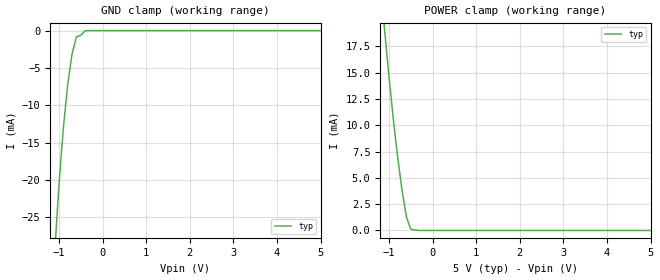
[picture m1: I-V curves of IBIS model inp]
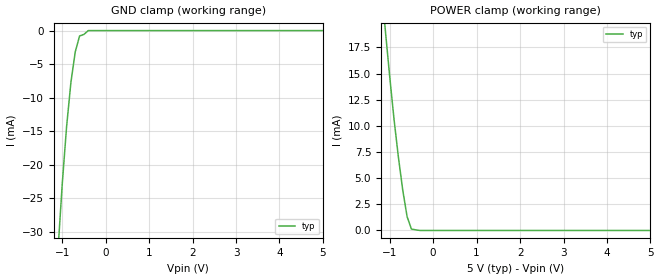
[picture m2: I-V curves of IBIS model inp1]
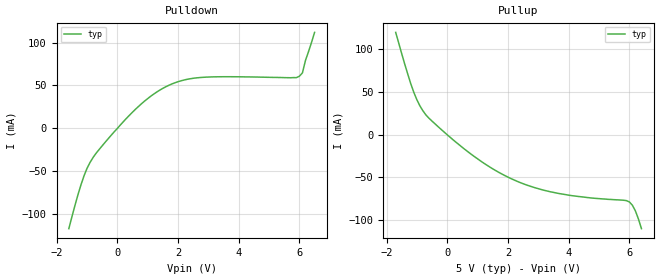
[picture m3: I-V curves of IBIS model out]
|Texas Instruments Incorporated
|SN65C1168 DUAL DIFFERENTIAL DRIVERS AND RECEIVERS
[IBIS Ver]   4.1
[File name]   sn65c1168.ibs
[Date]   02/08/2019
[File Rev]   1.0
[Source]
| Texas Instruments Incorporated.
| Analog-eLab Design Center, HPA
| 12500 TI Blvd
| Dallas, TX -75243
[Notes]   Revision History:
| Rev 1.0: 02/08/2019
| - Initial version of the model
| - IBIS model is done only for typical PVT corners
[Disclaimer]
| This model is designed as an aid for customers of Texas Instruments.
| TI and its licensors and suppliers make no warranties, either expressed
| or implied, with respect to this  model, including the warranties of
| merchantability or fitness for a particular purpose. The model is
| provided solely on an "as is" basis. The entire risk as to its quality
| and performance is with the customer.
| This model is subject to change without notice. Texas Instruments
| Incorporated is not responsible for updating this model.
|  Component SN65C1168N 16-Pin PDIP -N package
|  Part # SN65C1168N
[Component]   SN65C1168N
[Manufacturer]  TI
[Package]   |16 PDIP -N package
|   typ   min   max
R_pkg   0.05   NA   NA
L_pkg   1.0nH   NA   NA
C_pkg   0.2pF   NA   NA
[Pin]  signal_name   model_name   R_pin   L_pin   C_pin
1   1B   diff_in   NA   NA   NA
2   1A   diff_in   NA   NA   NA
3   1R   out   NA   NA   NA
4   1DE   inp1   NA   NA   NA
5   2R   out   NA   NA   NA
6   2A   diff_in   NA   NA   NA
7   2B   diff_in   NA   NA   NA
8   GND   gnd   NA   NA   NA
9   2D   inp   NA   NA   NA
10   2Y   diff_out   NA   NA   NA
11   2Z   diff_out   NA   NA   NA
12   2DE   inp1   NA   NA   NA
13   1Z   diff_out   NA   NA   NA
14   1Y   diff_out   NA   NA   NA
15   1D   inp   NA   NA   NA
16   VCC   power   NA   NA   NA
[Diff_pin]   inv_pin   vdiff   tdelay_typ   tdelay_min   tdelay_max
10   11   NA   NA   NA   NA
14   13   NA   NA   NA   NA
1   2   0.2   NA   NA   NA
6   7   0.2   NA   NA   NA
|  Component SN65C1168NS 16-Pin SOP -NS package
|  Part # SN65C1168NS
[Component]   SN65C1168NS
[Manufacturer]  TI
[Package]   |16 SOP -NS package
|   typ   min   max
R_pkg   0.05   NA   NA
L_pkg   1.0nH   NA   NA
C_pkg   0.2pF   NA   NA
[Pin]  signal_name   model_name   R_pin   L_pin   C_pin
1   1B   diff_in   NA   NA   NA
2   1A   diff_in   NA   NA   NA
3   1R   out   NA   NA   NA
4   1DE   inp1   NA   NA   NA
5   2R   out   NA   NA   NA
6   2A   diff_in   NA   NA   NA
7   2B   diff_in   NA   NA   NA
8   GND   gnd   NA   NA   NA
9   2D   inp   NA   NA   NA
10   2Y   diff_out   NA   NA   NA
11   2Z   diff_out   NA   NA   NA
12   2DE   inp1   NA   NA   NA
13   1Z   diff_out   NA   NA   NA
14   1Y   diff_out   NA   NA   NA
15   1D   inp   NA   NA   NA
16   VCC   power   NA   NA   NA
[Diff_pin]   inv_pin   vdiff   tdelay_typ   tdelay_min   tdelay_max
10   11   NA   NA   NA   NA
14   13   NA   NA   NA   NA
1   2   0.2   NA   NA   NA
6   7   0.2   NA   NA   NA
|  Component SN65C1168PW 16-Pin TSSOP -PW package
|  Part # SN65C1168PW
[Component]   SN65C1168PW
[Manufacturer]  TI
[Package]   |16 TSSOP -PW package
|   typ   min   max
R_pkg   0.05   NA   NA
L_pkg   1.0nH   NA   NA
C_pkg   0.2pF   NA   NA
[Pin]  signal_name   model_name   R_pin   L_pin   C_pin
1   1B   diff_in   NA   NA   NA
2   1A   diff_in   NA   NA   NA
3   1R   out   NA   NA   NA
4   1DE   inp1   NA   NA   NA
5   2R   out   NA   NA   NA
6   2A   diff_in   NA   NA   NA
7   2B   diff_in   NA   NA   NA
8   GND   gnd   NA   NA   NA
9   2D   inp   NA   NA   NA
10   2Y   diff_out   NA   NA   NA
11   2Z   diff_out   NA   NA   NA
12   2DE   inp1   NA   NA   NA
13   1Z   diff_out   NA   NA   NA
14   1Y   diff_out   NA   NA   NA
15   1D   inp   NA   NA   NA
16   VCC   power   NA   NA   NA
[Diff_pin]   inv_pin   vdiff   tdelay_typ   tdelay_min   tdelay_max
10   11   NA   NA   NA   NA
14   13   NA   NA   NA   NA
1   2   0.2   NA   NA   NA
6   7   0.2   NA   NA   NA
| Models and submodels in the file (5): inp (Input), inp1 (Input), out (Output), diff_out (Output), diff_in (Input)
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|   inp Model
[Model]   inp
Model_type   Input
Vinl = 0.8
Vinh = 2
|   typ   min   max
C_comp   4pF   NA   NA
| Where Nom  PVT is Nominal Process, 5.0V, 27C
[Voltage Range]   5.0   NA   NA
|Junction Temperature
[Temperature Range]   27   NA   NA
[Power Clamp Reference]   5.0   NA   NA
[GND Clamp Reference]   0   NA   NA
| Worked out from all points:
|   GND clamp passes 1 mA (typ) near -0.61 V on its own axis
|   POWER clamp passes 1 mA (typ) near -0.58 V on its own axis
[GND Clamp]
|   Voltage   I(typ)   I(min)   I(max)
-1.8V     -112.6mA   NA         NA
-1.1V     -29.86mA   NA         NA
-1V       -20.6mA    NA         NA
-900mV    -13.05mA   NA         NA
-800mV    -7.21mA    NA         NA
-700mV    -3.11mA    NA         NA
-600mV    -840uA     NA         NA
-500mV    -630uA     NA         NA
-400mV    0A         NA         NA
5V        0A         NA         NA
[POWER Clamp]
|   Voltage   I(typ)   I(min)   I(max)
-2.5V     100mA      NA         NA
-1.1V     18.99mA    NA         NA
-1V       14.61mA    NA         NA
-900mV    10.53mA    NA         NA
-800mV    6.92mA     NA         NA
-700mV    3.79mA     NA         NA
-600mV    1.28mA     NA         NA
-500mV    118uA      NA         NA
-300mV    0A         NA         NA
5V        0A         NA         NA
|   inp1 Model
[Model]   inp1
Model_type   Input
Vinl = 0.8
Vinh = 2
|   typ   min   max
C_comp   15pF   NA   NA
| Where Nom  PVT is Nominal Process, 5.0V, 27C
[Voltage Range]   5   NA   NA
|Junction Temperature
[Temperature Range]   27   NA   NA
[Power Clamp Reference]   5   NA   NA
[GND Clamp Reference]   0   NA   NA
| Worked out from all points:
|   GND clamp passes 1 mA (typ) near -0.61 V on its own axis
|   POWER clamp passes 1 mA (typ) near -0.57 V on its own axis
[GND Clamp]
|   Voltage   I(typ)   I(min)   I(max)
-1.8V     -119.6mA   NA         NA
-1.1V     -33.06mA   NA         NA
-1V       -22.94mA   NA         NA
-900mV    -14.38mA   NA         NA
-800mV    -7.735mA   NA         NA
-700mV    -3.175mA   NA         NA
-600mV    -800uA     NA         NA
-500mV    -574uA     NA         NA
-400mV    0A         NA         NA
5V        0A         NA         NA
[POWER Clamp]
|   Voltage   I(typ)   I(min)   I(max)
-2.7V     113.9mA    NA         NA
-1.1V     19.1mA     NA         NA
-1V       14.7mA     NA         NA
-900mV    10.6mA     NA         NA
-800mV    7mA        NA         NA
-700mV    3.85mA     NA         NA
-600mV    1.32mA     NA         NA
-500mV    132uA      NA         NA
-300mV    0A         NA         NA
5V        0A         NA         NA
|   out Model
[Model]   out
Model_type   Output
Polarity   Non-Inverting
Vmeas = 2.5
Vref = 0
Cref = 2pF
Rref = 100000
|   typ   min   max
C_comp   15pF   NA   NA
| Where Nom  PVT is Nominal Process, 5V, 27C
[Voltage Range]   5   NA   NA
|Junction Temperature
[Temperature Range]   27   NA   NA
[Pullup Reference]   5   NA   NA
[Pulldown Reference]   0   NA   NA
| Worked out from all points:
|   slope of the pulldown table from 0 to 0.75 V, typ, clamps not added: 27.4 ohm
|   slope of the pullup table from 0 to 0.75 V, typ, clamps not added: 34.5 ohm
[Pulldown]
|   Voltage   I(typ)   I(min)   I(max)
-1.6V     -117.1mA   NA         NA
-1.2V     -66.06mA   NA         NA
-900mV    -39.82mA   NA         NA
-700mV    -29.1mA    NA         NA
100mV     3.868mA    NA         NA
1V        34.6mA     NA         NA
1.7V      50.15mA    NA         NA
2.5V      58.29mA    NA         NA
5.9V      59.05mA    NA         NA
6.1V      64.64mA    NA         NA
6.2V      79.19mA    NA         NA
6.5V      111.8mA    NA         NA
[Pullup]
|   Voltage   I(typ)   I(min)   I(max)
-1.7V     119.8mA    NA         NA
-1.2V     59.3mA     NA         NA
-1V       40.7mA     NA         NA
-900mV    33.54mA    NA         NA
-600mV    19.12mA    NA         NA
500mV     -15.07mA   NA         NA
1.7V      -44.26mA   NA         NA
2.7V      -60.06mA   NA         NA
4V        -70.94mA   NA         NA
6V        -78.85mA   NA         NA
6.2V      -89.36mA   NA         NA
6.4V      -110.2mA   NA         NA
[Ramp]
R_load = 50
|   typ   min   max
dV/dt_r   1.8/0.25e-8   NA   NA
dV/dt_f   1.8/2.13e-9   NA   NA
